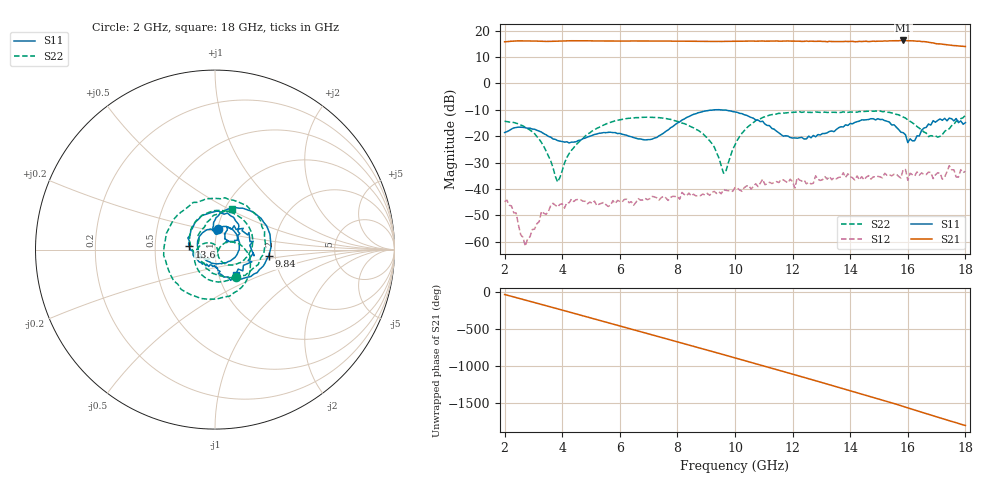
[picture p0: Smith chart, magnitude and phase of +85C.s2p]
!Agilent Technologies,N5230A,MY45001466,A.07.50.67
!Agilent N5230A: A.07.50.67
!Date: Monday, February 09, 2026 16:27:56
!Correction: S11(Full 2 Port(1,2))
!S21(Full 2 Port(1,2))
!S12(Full 2 Port(1,2))
!S22(Full 2 Port(1,2))
!S2P File: Measurements: S11, S21, S12, S22:
# Hz S  dB  R 50
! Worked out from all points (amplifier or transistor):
!   201 points, 2 GHz to 18 GHz, reference 50 ohm
!   highest |S21| = 16.3 dB at 15.84 GHz (marker M1)
!   |S21| within 3 dB of that: start of sweep to end of sweep
!   unconditionally stable (mu >= 1): start of sweep to end of sweep
!   at 4.64 GHz: K = 12.27, MAG = 16.2 dB, |S12| = -44.1 dB
!   at 10 GHz: K = 6.85, MAG = 16.4 dB, |S12| = -39.5 dB
!   at 18 GHz: K = 4.20, MAG = 14.5 dB, |S12| = -33.3 dB
!   S11 on the Smith chart (normalised r, x): 2 GHz: 1.00, +0.24; 9.84 GHz: 1.85, -0.14; 13.6 GHz: 0.75, +0.03; 18 GHz: 1.20, -0.35
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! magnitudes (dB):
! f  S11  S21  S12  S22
! 2 GHz  -18.6  15.8  -44.8  -14.3
! 2.4 GHz  -16.7  16.1  -49.1  -15.0
! 2.72 GHz  -16.8  16.1  -61.7  -16.7
! 3.28 GHz  -18.4  16.0  -48.5  -22.4
! 3.84 GHz  -21.6  16.0  -46.8  -37.4
! 4.16 GHz  -22.1  16.2  -45.2  -28.1
! 4.72 GHz  -20.9  16.2  -44.6  -20.9
! 5.84 GHz  -18.6  16.1  -45.5  -14.1
! 7.36 GHz  -19.9  16.0  -44.2  -13.0
! 8.88 GHz  -10.7  15.9  -41.9  -19.0
! 9.6 GHz  -10.1  15.9  -40.2  -34.0
! 9.84 GHz  -10.4  15.9  -40.8  -27.7
! 10 GHz  -10.8  16.0  -39.5  -23.3
! 10.96 GHz  -14.3  16.1  -36.3  -12.9
! 11.68 GHz  -20.0  16.0  -36.5  -11.3
! 12.72 GHz  -19.7  16.0  -37.8  -11.0
! 13.6 GHz  -16.8  15.9  -35.6  -11.1
! 15.36 GHz  -14.6  16.1  -34.6  -11.0
! 15.84 GHz  -18.7  16.3  -32.6  -12.8
! 16.24 GHz  -21.7  16.1  -35.0  -15.6
! 17.04 GHz  -14.0  15.0  -33.9  -20.4
! 18 GHz  -14.9  14.0  -33.3  -12.1
